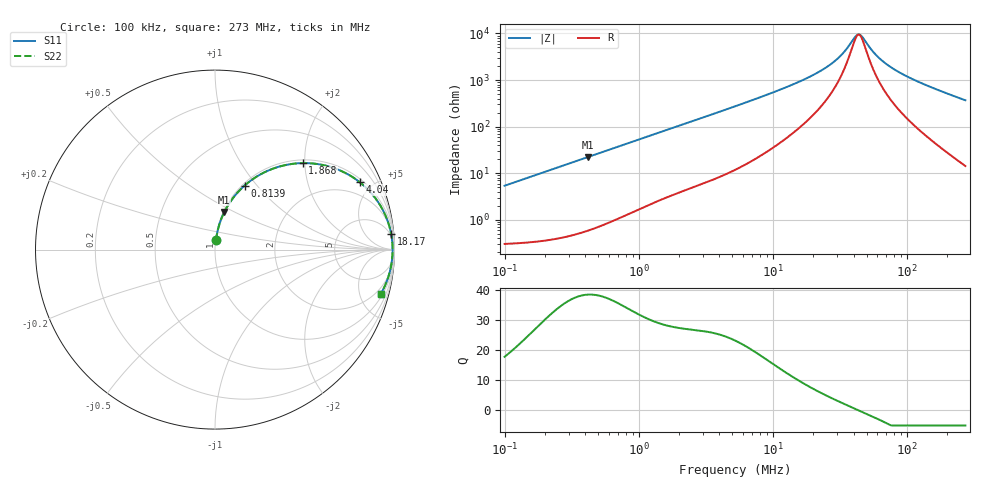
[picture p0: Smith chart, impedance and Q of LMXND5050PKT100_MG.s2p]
! LMXND5050PKT100_MG  S-PARAMETER MODEL  ( General Type )
! Model Generated by TAIYO YUDEN Corporation (http://www.ty-top.com)
! Version 1.0
! TAIYO YUDEN Control No. 191023NI43SB-FBB
! Copyright(c) 2019 TAIYO YUDEN CO.,LTD. All Rights Reserved.
! Product Description (link to TY-COMPAS)
! https://ds.yuden.co.jp/TYCOMPAS/or/detail?pn=LMXND5050PKT100MMG&u=M
! Products Name : Inductors
! Characteristics :
!  Inductance : 10 uH , SRF(min) : 27 MHz , DC Resistance(max) : 0.24 Ohm
!  Rated Current : Saturation :1400 mA , Temp Rise : 1050 mA
!  Case Size : 4.9 x 4.9 / 0.193 x 0.193 [mm/inch] , Thickness : 1.4 / 0.055 [mm/inch]
!  (Conditions: Temperature = 25 degC , DC Bias Current/Voltage = 0A / 0V)
! External Node Assignments :
!  1  o---GGG---o  2
! GND o---------o GND
! Frequency Range : 0.1MHz  -  272.98108MHz  [ 402 STEP ]
# MHz S RI R 50
! Freq[MHz].  S11 Real  S11 Imag  S21 Real  S21 Imag  S12 Real  S12 Imag  S22 Real  S22 Imag
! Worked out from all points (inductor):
!   401 points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, 100 kHz to 273 MHz, reference 50 ohm
!   read as one part in series: L = 8.54 uH near 104 kHz
!   highest Q = 38.3 at 415.4 kHz (marker M1), where L = 8.51 uH
!   self-resonance near 43.37 MHz
!   S11 on the Smith chart (normalised r, x): 100 kHz: 1.01, +0.11; 813.9 kHz: 1.03, +0.86; 1.868 MHz: 1.07, +1.95; 4.04 MHz: 1.17, +4.19; 18.17 MHz: 4, +22; 273 MHz: 1.28, -7.33
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0.1  0.00586 0.0532  0.9941 -0.0532  0.9941 -0.0532  0.00586 0.0532
0.376316  0.0436 0.1915  0.9564 -0.1915  0.9564 -0.1915  0.0436 0.1915
0.415436  0.052 0.2093  0.948 -0.2093  0.948 -0.2093  0.052 0.2093
0.813908  0.1648 0.3565  0.8352 -0.3565  0.8352 -0.3565  0.1648 0.3565
1.416134  0.3615 0.4634  0.6385 -0.4634  0.6385 -0.4634  0.3615 0.4634
1.867966  0.4889 0.482  0.5111 -0.482  0.5111 -0.482  0.4889 0.482
2.666828  0.6525 0.4577  0.3475 -0.4577  0.3475 -0.4577  0.6525 0.4577
4.040099  0.8053 0.3765  0.1947 -0.3765  0.1947 -0.3765  0.8053 0.3765
5.329134  0.8748 0.3099  0.1252 -0.3099  0.1252 -0.3099  0.8748 0.3099
10.64923  0.9604 0.1637  0.0396 -0.1637  0.0396 -0.1637  0.9604 0.1637
18.16591  0.9816 0.0864  0.0184 -0.0864  0.0184 -0.0864  0.9816 0.0864
19.66158  0.9832 0.0771  0.0168 -0.0771  0.0168 -0.0771  0.9832 0.0771
24.92886  0.9867 0.0516  0.0133 -0.0516  0.0133 -0.0516  0.9867 0.0516
29.78622  0.9883 0.0343  0.0117 -0.0343  0.0117 -0.0343  0.9883 0.0343
34.20958  0.9891 0.0216  0.0109 -0.0216  0.0109 -0.0216  0.9891 0.0216
40.87528  0.9896 0.00584  0.0104 -0.00584  0.0104 -0.00584  0.9896 0.00584
43.37423  0.9896 0.000636  0.0104 -0.000636  0.0104 -0.000636  0.9896 0.000636
46.9454  0.9896 -0.0063  0.0104 0.0063  0.0104 0.0063  0.9896 -0.0063
59.52193  0.9889 -0.0275  0.0111 0.0275  0.0111 0.0275  0.9889 -0.0275
73.9896  0.9873 -0.0482  0.0127 0.0482  0.0127 0.0482  0.9873 -0.0482
123.7426  0.9779 -0.1074  0.0221 0.1074  0.0221 0.1074  0.9779 -0.1074
272.9811  0.9225 -0.2487  0.0775 0.2487  0.0775 0.2487  0.9225 -0.2487
